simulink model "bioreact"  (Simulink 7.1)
settings: Solver=ode45  SolverMode=SingleTasking  StartTime=0.0  StopTime=inf  RelTol=1e-3  AbsTol=1e-6
PostLoadFcn:
  | arlab3_postloadfcn
StartFcn:
  | arlab3_startfcn
StopFcn:
  | arlab3_stopfcn
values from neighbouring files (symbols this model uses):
  h = findobj(gcf,'Type','axes')    [suptitle.m]    (also in arlab3_postloadfcn.m = 0.1)
  y = u(2)    [reg.m]    (also in sevalmode.m)
undefined symbols (not defined in the file or in its folder): w

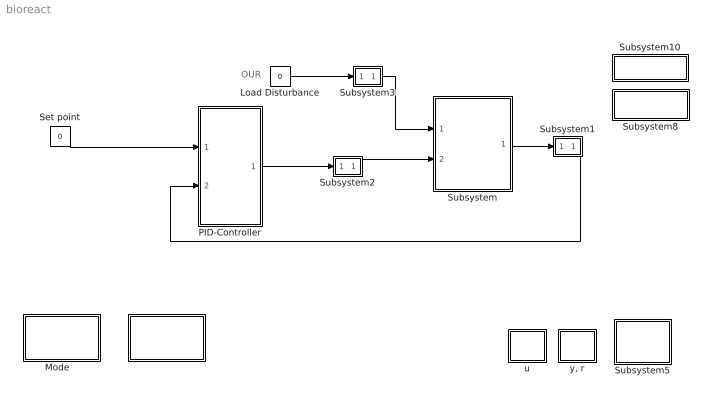
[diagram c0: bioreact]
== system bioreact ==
  note: OUR
  "    " : Subsystem
  Load Disturbance : Constant  Value=0
  "Mode   " : Subsystem
  PID-Controller : Subsystem
  Set point : Constant  Value=0
  Subsystem : Subsystem
  Subsystem1 : Subsystem  mask{vname=y}
      mask prompts: vname "Variable name"
      mask init:
      | parent = get_param(gcb,'Parent');
      | name = get_param(gcb,'Name');
      | set_param([parent '/' name '/Goto'],'GotoTag',vname)
  Subsystem10 : Subsystem
  Subsystem2 : Subsystem  mask{vname=u}
      mask prompts: vname "Variable name"
      mask init:
      | parent = get_param(gcb,'Parent');
      | name = get_param(gcb,'Name');
      | set_param([parent '/' name '/Goto'],'GotoTag',vname)
  Subsystem3 : Subsystem  mask{vname=w}
      mask prompts: vname "Variable name"
      mask init:
      | parent = get_param(gcb,'Parent');
      | name = get_param(gcb,'Name');
      | set_param([parent '/' name '/Goto'],'GotoTag',vname)
  Subsystem5 : Subsystem
  Subsystem8 : Subsystem
  u : Subsystem
  "y, r" : Subsystem
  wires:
  Set point/1 -> PID-Controller/1(In1)
  Load Disturbance/1 -> Subsystem3/1(In)
  PID-Controller/1(Out2) -> Subsystem2/1(In)
  Subsystem1/1(Out) -> PID-Controller/2(In2)
  Subsystem3/1(Out) -> Subsystem/1(In1)
  Subsystem2/1(Out) -> Subsystem/2(In2)
  Subsystem/1(Out1) -> Subsystem1/1(In)

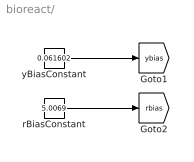
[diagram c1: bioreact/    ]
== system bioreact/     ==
  rBiasConstant : Constant  Value=5.0069
  yBiasConstant : Constant  Value=0.061602
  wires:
  yBiasConstant/1 -> [ybias]
  rBiasConstant/1 -> [rbias]

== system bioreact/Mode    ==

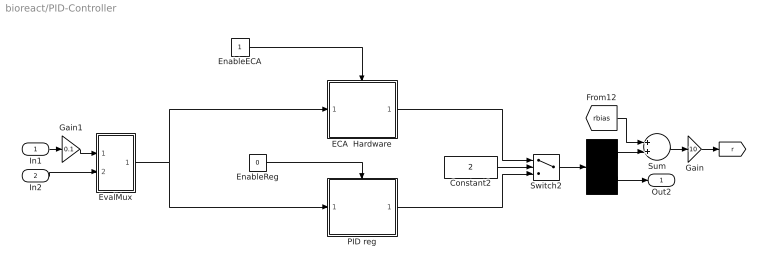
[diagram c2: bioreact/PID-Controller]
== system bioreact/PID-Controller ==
  In1 : Inport
  In2 : Inport  Port=2
  " " : Demux  Outputs=2
  Constant2 : Constant  Value=2
  ECA  Hardware : Subsystem
  EnableECA : Constant
  EnableReg : Constant  Value=0
  EvalMux : Subsystem
  Gain : Gain  Gain=10
  Gain1 : Gain  Gain=0.1
  PID reg : Subsystem
  Sum : Sum
  Switch2 : Switch  Threshold=2
  Out2 : Outport
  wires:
  Constant2/1 -> Switch2/2
  ECA  Hardware/1("[ r  u ]") -> Switch2/1
  PID reg/1("[ r u ]") -> Switch2/3
  Switch2/1 -> " "/1
  " "/2 -> Out2/1
  " "/1 -> Sum/2
  [rbias] -> Sum/1
  EnableECA/1 -> ECA  Hardware/Enable
  EnableReg/1 -> PID reg/Enable
  In2/1 -> EvalMux/2(In2)
  EvalMux/1(Out1) -> ECA  Hardware/1("[ r  y ]"), PID reg/1("[ r y ]")
  In1/1 -> Gain1/1
  Gain1/1 -> EvalMux/1(In1)
  Sum/1 -> Gain/1
  Gain/1 -> [r]

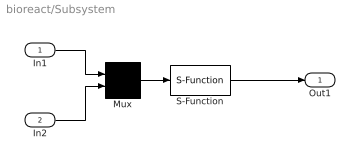
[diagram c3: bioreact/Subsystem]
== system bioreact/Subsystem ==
  In1 : Inport
  In2 : Inport  Port=2
  Mux : Mux  Inputs=2
  S-Function : S-Function  FunctionName=bioreactor  EnableBusSupport=off
  Out1 : Outport
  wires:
  In1/1 -> Mux/1
  In2/1 -> Mux/2
  Mux/1 -> S-Function/1
  S-Function/1 -> Out1/1

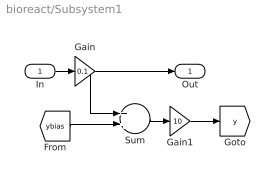
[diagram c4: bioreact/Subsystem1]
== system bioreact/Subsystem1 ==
  In : Inport
  Gain : Gain  Gain=0.1
  Gain1 : Gain  Gain=10
  Sum : Sum
  Out : Outport
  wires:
  [ybias] -> Sum/2
  In/1 -> Gain/1
  Gain/1 -> Out/1, Sum/1
  Sum/1 -> Gain1/1
  Gain1/1 -> [y]

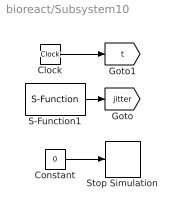
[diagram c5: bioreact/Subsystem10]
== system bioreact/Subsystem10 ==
  Clock : Clock
  Constant : Constant  Value=0
  S-Function1 : S-Function  FunctionName=realtimer  Parameters=h  EnableBusSupport=off
  Stop Simulation : Stop
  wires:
  Constant/1 -> Stop Simulation/1
  S-Function1/1 -> [jitter]
  Clock/1 -> [t]

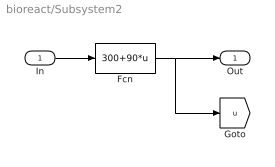
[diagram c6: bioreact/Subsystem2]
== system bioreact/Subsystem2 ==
  In : Inport
  Fcn : Fcn  Expr=300+90*u
  Out : Outport
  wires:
  In/1 -> Fcn/1
  Fcn/1 -> Out/1, [u]

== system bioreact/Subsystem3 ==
  In : Inport
  Out : Outport
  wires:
  In/1 -> Out/1, [w]

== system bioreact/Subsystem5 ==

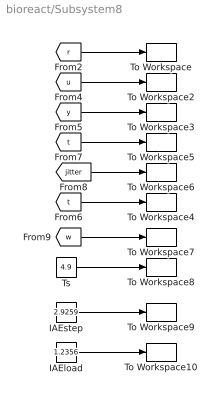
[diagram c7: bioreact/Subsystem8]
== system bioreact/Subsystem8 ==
  IAEload : Constant  Value=1.2356
  IAEstep : Constant  Value=2.9259
  To Workspace : ToWorkspace  VariableName=r  SampleTime=h  SaveFormat=Array
  To Workspace10 : ToWorkspace  VariableName=IAEload  SampleTime=h  SaveFormat=Array
  To Workspace2 : ToWorkspace  VariableName=u  SampleTime=h  SaveFormat=Array
  To Workspace3 : ToWorkspace  VariableName=y  SampleTime=h  SaveFormat=Array
  To Workspace4 : ToWorkspace  VariableName=tc  SampleTime=h  SaveFormat=Array
  To Workspace5 : ToWorkspace  VariableName=t  SampleTime=h  SaveFormat=Array
  To Workspace6 : ToWorkspace  VariableName=jitter  SampleTime=h  SaveFormat=Array
  To Workspace7 : ToWorkspace  VariableName=w  SampleTime=h  SaveFormat=Array
  To Workspace8 : ToWorkspace  VariableName=Ts  SampleTime=h  SaveFormat=Array
  To Workspace9 : ToWorkspace  VariableName=IAEstep  SampleTime=h  SaveFormat=Array
  Ts : Constant  Value=4.9
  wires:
  [t] -> To Workspace4/1
  [t] -> To Workspace5/1
  [jitter] -> To Workspace6/1
  [y] -> To Workspace3/1
  [u] -> To Workspace2/1
  [r] -> To Workspace/1
  [w] -> To Workspace7/1
  Ts/1 -> To Workspace8/1
  IAEstep/1 -> To Workspace9/1
  IAEload/1 -> To Workspace10/1

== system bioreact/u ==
  u : Scope
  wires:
  [u] -> u/1

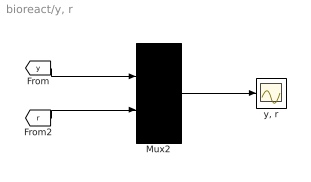
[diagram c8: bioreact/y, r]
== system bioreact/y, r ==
  Mux2 : Mux  Inputs=2
  "y, r" : Scope
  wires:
  [r] -> Mux2/2
  [y] -> Mux2/1
  Mux2/1 -> "y, r"/1

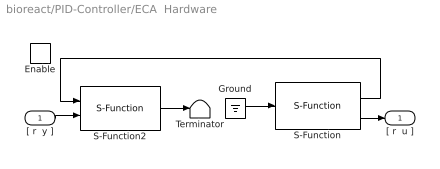
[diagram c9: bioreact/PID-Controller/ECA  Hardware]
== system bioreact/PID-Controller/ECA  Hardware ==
  "[ r  y ]" : Inport
  Enable : EnablePort
  Ground : Ground
  S-Function : S-Function  FunctionName=analogin  Parameters=h [1 0]  EnableBusSupport=off
  S-Function2 : S-Function  FunctionName=analogout  Parameters=h [1 0]  EnableBusSupport=off
  Terminator : Terminator
  "[ r  u ]" : Outport  InitialOutput=0
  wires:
  Ground/1 -> S-Function/1
  S-Function2/1 -> Terminator/1
  S-Function/1 -> S-Function2/1
  S-Function/2 -> "[ r  u ]"/1
  "[ r  y ]"/1 -> S-Function2/2

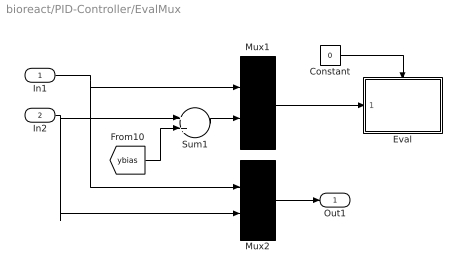
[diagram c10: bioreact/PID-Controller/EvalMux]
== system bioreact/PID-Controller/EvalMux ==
  In1 : Inport
  In2 : Inport  Port=2
  Constant : Constant  Value=0
  Eval : Subsystem
  Mux1 : Mux  Inputs=2
  Mux2 : Mux  Inputs=2
  Sum1 : Sum
  Out1 : Outport  InitialOutput=0
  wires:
  Mux2/1 -> Out1/1
  Sum1/1 -> Mux1/2
  [ybias] -> Sum1/2
  In2/1 -> Mux2/2, Sum1/1
  Mux1/1 -> Eval/1(In1)
  Constant/1 -> Eval/Enable
  In1/1 -> Mux2/1, Mux1/1

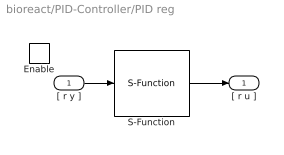
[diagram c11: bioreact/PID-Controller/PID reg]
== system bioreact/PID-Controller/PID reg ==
  "[ r y ]" : Inport
  Enable : EnablePort
  S-Function : S-Function  FunctionName=reg  Parameters=h  EnableBusSupport=off
  "[ r u ]" : Outport
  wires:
  S-Function/1 -> "[ r u ]"/1
  "[ r y ]"/1 -> S-Function/1

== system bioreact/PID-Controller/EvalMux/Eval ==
  In1 : Inport
  Enable : EnablePort
  S-eval : S-Function  FunctionName=sevalmode  Parameters=h,1,1,'bioreact'  EnableBusSupport=off
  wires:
  In1/1 -> S-eval/1
